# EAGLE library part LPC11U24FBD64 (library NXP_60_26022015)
32-bit ARM Cortex-M0 microcontroller; up to 32 kB flash; up to 10 kB SRAM and 4 kB EEPROM; USB device; USART The LPC11U2x are an ARM Cortex-M0 based, low-cost 32-bit MCU family, designed for 8/16-bit microcontroller applications, offering performance, low power, simple instruction set and memory addressing together with reduced code size compared to existing 8/16-bit architectures. The LPC11U2x operate at CPU frequencies of up to 50 MHz. Equipped with a highly flexible and configurable Full-Speed USB 2.0 device controller, the LPC11U2x brings unparalleled design flexibility and seamless integration to today’s demanding connectivity solutions. The peripheral complement of the LPC11U2x includes up to 32 kB of flash memory, up to 10 kB of SRAM data memory and 4 kB EEPROM, one Fast-mode Plus I 2 C-bus interface, one RS-485/EIA-485 USART with support for synchronous mode and smart card interface, two SSP interfaces, four general-purpose counter/timers, a 10-bit ADC (Analog-to-Digital Converter), and up to 54 general-purpose I/O pins. AAL Eindhoven MK
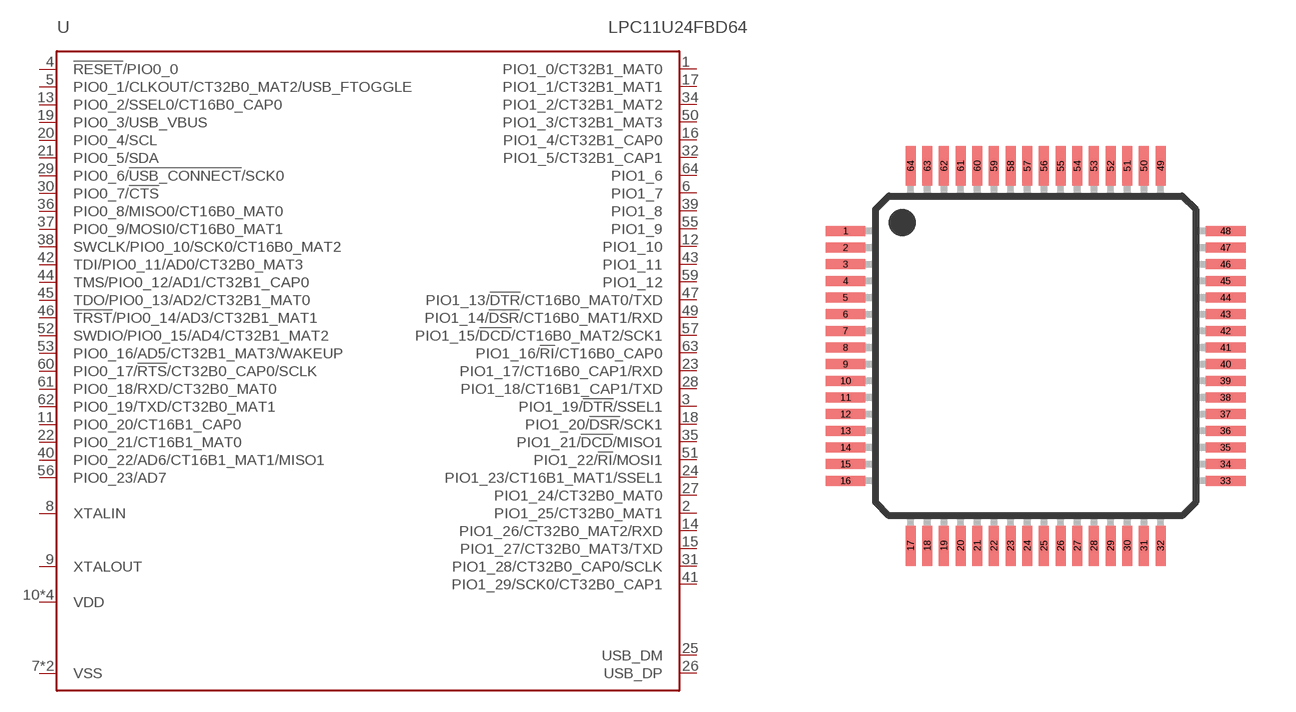
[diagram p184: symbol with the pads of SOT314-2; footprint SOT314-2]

Designator prefix U

## LPC11U24FBD64/401 (EEPROM: 4kB; FLASH: 32kB; GPIO: 54; SRAM: 8kB; USB_SRAM: 2kB)  [SOT314-2]
1  PIO1_0/CT32B1_MAT0
2  PIO1_25/CT32B0_MAT1
3  PIO1_19/!DTR!/SSEL1
4  !RESET!/PIO0_0
5  PIO0_1/CLKOUT/CT32B0_MAT2/USB_FTOGGLE
6  PIO1_7
7  VSS  pwr
8  XTALIN  in
9  XTALOUT  out
10  VDD  pwr
11  PIO0_20/CT16B1_CAP0
12  PIO1_10
13  PIO0_2/SSEL0/CT16B0_CAP0
14  PIO1_26/CT32B0_MAT2/RXD
15  PIO1_27/CT32B0_MAT3/TXD
16  PIO1_4/CT32B1_CAP0
17  PIO1_1/CT32B1_MAT1
18  PIO1_20/!DSR!/SCK1
19  PIO0_3/USB_VBUS
20  PIO0_4/SCL
21  PIO0_5/SDA
22  PIO0_21/CT16B1_MAT0
23  PIO1_17/CT16B0_CAP1/RXD
24  PIO1_23/CT16B1_MAT1/SSEL1
25  USB_DM
26  USB_DP
27  PIO1_24/CT32B0_MAT0
28  PIO1_18/CT16B1_CAP1/TXD
29  PIO0_6/!USB_CONNECT!/SCK0
30  PIO0_7/!CTS!
31  PIO1_28/CT32B0_CAP0/SCLK
32  PIO1_5/CT32B1_CAP1
33  VDD  pwr
34  PIO1_2/CT32B1_MAT2
35  PIO1_21/!DCD!/MISO1
36  PIO0_8/MISO0/CT16B0_MAT0
37  PIO0_9/MOSI0/CT16B0_MAT1
38  SWCLK/PIO0_10/SCK0/CT16B0_MAT2
39  PIO1_8
40  PIO0_22/AD6/CT16B1_MAT1/MISO1
41  PIO1_29/SCK0/CT32B0_CAP1
42  TDI/PIO0_11/AD0/CT32B0_MAT3
43  PIO1_11
44  TMS/PIO0_12/AD1/CT32B1_CAP0
45  TDO/PIO0_13/AD2/CT32B1_MAT0
46  !TRST!/PIO0_14/AD3/CT32B1_MAT1
47  PIO1_13/!DTR!/CT16B0_MAT0/TXD
48  VDD  pwr
49  PIO1_14/!DSR!/CT16B0_MAT1/RXD
50  PIO1_3/CT32B1_MAT3
51  PIO1_22/!RI!/MOSI1
52  SWDIO/PIO0_15/AD4/CT32B1_MAT2
53  PIO0_16/AD5/CT32B1_MAT3/WAKEUP
54  VSS  pwr
55  PIO1_9
56  PIO0_23/AD7
57  PIO1_15/!DCD!/CT16B0_MAT2/SCK1
58  VDD  pwr
59  PIO1_12
60  PIO0_17/!RTS!/CT32B0_CAP0/SCLK
61  PIO0_18/RXD/CT32B0_MAT0
62  PIO0_19/TXD/CT32B0_MAT1
63  PIO1_16/!RI!/CT16B0_CAP0
64  PIO1_6

## Footprint SOT314-2 (pad centres in mm)
SOT314-2 LQFP64: plastic low profile quad flat package; 64 leads; body 10 x 10 x 1.4 mm JEDEC: MS-026 IEC: 136E10
smd 1.2 x 0.3: 1 -5.7,3.75; 2 -5.7,3.25; 3 -5.7,2.75; 4 -5.7,2.25; 5 -5.7,1.75; 6 -5.7,1.25; 7 -5.7,0.75; 8 -5.7,0.25; 9 -5.7,-0.25; 10 -5.7,-0.75; 11 -5.7,-1.25; 12 -5.7,-1.75; 13 -5.7,-2.25; 14 -5.7,-2.75; 15 -5.7,-3.25; 16 -5.7,-3.75; 33 5.7,-3.75; 34 5.7,-3.25; 35 5.7,-2.75; 36 5.7,-2.25; 37 5.7,-1.75; 38 5.7,-1.25; 39 5.7,-0.75; 40 5.7,-0.25; 41 5.7,0.25; 42 5.7,0.75; 43 5.7,1.25; 44 5.7,1.75; 45 5.7,2.25; 46 5.7,2.75; 47 5.7,3.25; 48 5.7,3.75
smd 0.3 x 1.2: 17 -3.75,-5.7; 18 -3.25,-5.7; 19 -2.75,-5.7; 20 -2.25,-5.7; 21 -1.75,-5.7; 22 -1.25,-5.7; 23 -0.75,-5.7; 24 -0.25,-5.7; 25 0.25,-5.7; 26 0.75,-5.7; 27 1.25,-5.7; 28 1.75,-5.7; 29 2.25,-5.7; 30 2.75,-5.7; 31 3.25,-5.7; 32 3.75,-5.7; 49 3.75,5.7; 50 3.25,5.7; 51 2.75,5.7; 52 2.25,5.7; 53 1.75,5.7; 54 1.25,5.7; 55 0.75,5.7; 56 0.25,5.7; 57 -0.25,5.7; 58 -0.75,5.7; 59 -1.25,5.7; 60 -1.75,5.7; 61 -2.25,5.7; 62 -2.75,5.7; 63 -3.25,5.7; 64 -3.75,5.7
